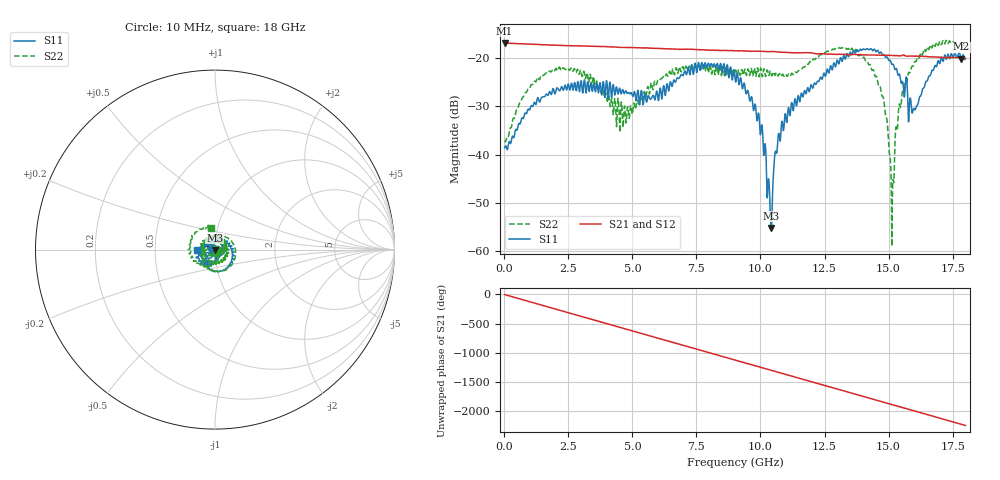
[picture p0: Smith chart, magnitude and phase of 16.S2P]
!Agilent Technologies,E5071C,MY46316741,A.11.02
!Date: Fri May 06 15:20:13 2022
!Data & Calibration Information:
!Freq	S11:SOLT2(ON)	S21:SOLT2(ON)	S12:SOLT2(ON)	S22:SOLT2(ON)
!PortZ  Port1:50+j0  Port2:50+j0
!Above PortZ is port z conversion or system Z0 setting when saving the data.
!When reading, reference impedance value at option line is always used.
# Hz S dB R 50
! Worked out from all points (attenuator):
!   1800 points, 10 MHz to 18 GHz, reference 50 ohm
!   highest |S21| = -16.83 dB at 10 MHz (marker M1); lowest = -20.1 dB at 17.84 GHz (marker M2)
!   lowest |S11| = -55.2 dB at 10.42 GHz (marker M3), VSWR 1.00, Z = 49.9 - j0.148 ohm
!   |S11| at or under -10 dB: start of sweep to end of sweep
!   |S22| runs from -59.0 to -16.3 dB; largest |S21 - S12| = 0.0084
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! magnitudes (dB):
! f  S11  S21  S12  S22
! 10 MHz  -38.6  -16.8  -16.8  -37.1
! 1.24 GHz  -29.5  -17.1  -17.1  -24.8
! 3.01 GHz  -24.9  -17.4  -17.5  -23.1
! 4.57 GHz  -27.3  -17.7  -17.8  -29.1
! 6.01 GHz  -28.8  -18.0  -18.0  -24.5
! 7.64 GHz  -22.5  -18.2  -18.3  -21.5
! 9.01 GHz  -24.2  -18.5  -18.5  -22.7
! 9.99 GHz  -35.7  -18.6  -18.6  -22.4
! 10.42 GHz  -55.2  -18.6  -18.7  -23.3
! 10.63 GHz  -39.7  -18.7  -18.7  -23.0
! 10.9 GHz  -35.0  -18.8  -18.8  -23.6
! 12.01 GHz  -25.9  -18.9  -19.0  -20.7
! 14.1 GHz  -18.2  -19.3  -19.4  -20.5
! 14.73 GHz  -18.9  -19.3  -19.4  -27.6
! 15.01 GHz  -20.5  -19.4  -19.4  -38.6
! 15.16 GHz  -21.2  -19.5  -19.4  -46.4
! 15.33 GHz  -22.5  -19.5  -19.5  -34.9
! 15.47 GHz  -24.5  -19.5  -19.5  -30.2
! 15.99 GHz  -30.4  -19.5  -19.6  -21.1
! 17 GHz  -21.1  -19.8  -19.9  -16.5
! 17.84 GHz  -20.4  -20.1  -20.1  -17.3
! 18 GHz  -20.2  -20.0  -20.2  -18.4
